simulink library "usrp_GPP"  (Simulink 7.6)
settings: Solver=ode45  SolverMode=SingleTasking  StartTime=0.0  StopTime=10.0  RelTol=1e-3
undefined symbols (not defined in the file or in its folder): Bit, Channels, Complex, Disabled, INT16, kB, kSps, Mbit, N, S, s, zwei

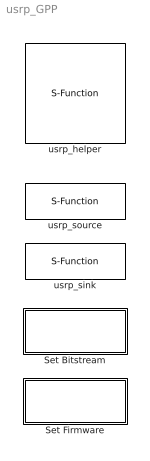
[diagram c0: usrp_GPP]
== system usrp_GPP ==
  Set Bitstream : Subsystem  mask{bitfile=zwei.rbf}
      mask prompts: bitfile "FPGA Bitfile"
  Set Firmware : Subsystem  mask{bitfile=zwei.rbf}
      mask prompts: bitfile "FPGA Bitfile"
  usrp_helper : S-Function  FunctionName=usrp_helper  EnableBusSupport=off  mask(USRP Helper){usrp_number=0, serial_number=S/N: 4556d9c1., daughterboards_rx=RX A: Flex 2400 Rx, RX B: WBX NG RX,, daughterboards_tx=TX A: Flex 2400 Tx, TX B: WBX NG TX., usb_block_size=0, usb_nblocks=0, firmware=C:\\Users\\nagel\\Documents\\sff_sdr\\Simulink-USRP\\simulink-usrp_2.1.0\\firmware\\rev4\\std.ihx, bitstream=C:\\Users\\nagel\\Documents\\sff_sdr\\Simulink-USRP\\simulink-usrp_2.1.0\\firmware\\rev4\\std_2rxhb_2tx.rbf, sample_time_factor=1}
      mask prompts: usrp_number "USRP Board Number:"; serial_number "Serial Number:"; daughterboards_rx "RX Daughterboards:"; daughterboards_tx "TX Daughterboards:"; usb_block_size "USB Block Size:"; usb_nblocks "USB Number of Blocks:"; firmware "Firmware Filename:"; bitstream "FPGA Bitstream Filename:"; sample_time_factor "Sample Time Factor:"
      mask help: Use this block to set common settings for a USRP device.
      mask init:
      | % Set default bitstream and firmware if not specified yet
      | bitstream_std_path = fullfile(usrpGetFirmwarePath(),'rev4','std_2rxhb_2tx.rbf');
      | firmware_std_path = fullfile(usrpGetFirmwarePath(),'rev4','std.ihx');
      | 
      | if strcmp(get_param(gcb,'firmware'),'')
      |     set_param(gcb,'firmware',firmware_std_path)
      | end
      |     
      | if strcmp(get_param(gcb,'bitstream'),'')
      |     set_param(gcb,'bitstream',bitstream_std_path)
      | end
  usrp_sink : S-Function  FunctionName=usrp_sink  Parameters=usrp_number,decimation,sample_width,vector_length,sideA_subdev1_datatype,sideA_subdev1_frequency,sideA_subdev1_frequency_port,sideA_subdev1_gain,sideB_subdev1_datatype,sideB_subdev1_frequency,sideB_subdev1_frequency_port,sideB_subdev1_gain, usrp_helper('GetParam', 'sample_time_factor'), usrp_helper('GetParam', 'usb_block_size'), usrp_helper('GetParam', 'usb_nblocks'), usrp_helper('GetParam', 'firm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  EnableBusSupport=off  mask(USRP Sink){usrp_number=0, serial_number=Unknown (USRP Board #0 not found)., decimation=512, sample_width=16 Bit, sampling_rate_and_bandwidth=1 Channels: 250 kSps, 976.563 kB/s, 7.62939 Mbit/s., vector_length=1024, sideA_subdev1_tab_=0, sideA_subdev1_subdevice=Unknown (USRP Board #0 not found)., sideA_subdev1_datatype=INT16 Complex, sideA_subdev1_frequency_range=Unknown., sideA_subdev1_frequency_port=off, sideA_subdev1_frequency=0, sideA_subdev1_gain_range=Unknown., sideA_subdev1_gain=0, sideB_subdev1_tab_=0, sideB_subdev1_subdevice=Unknown (USRP Board #0 not found)., sideB_subdev1_datatype=Disabled, sideB_subdev1_frequency_range=Unknown., sideB_subdev1_frequency_port=off, sideB_subdev1_frequency=0, sideB_subdev1_gain_range=Unknown., sideB_subdev1_gain=0}
      mask prompts: usrp_number "USRP Board Number:"; serial_number "Serial Number:"; decimation "Interpolation Factor:"; sample_width "Sample Width:"; sampling_rate_and_bandwidth "Effective Sampling Rate and Bandwidth:"; vector_length "Vector length:"; sideA_subdev1_tab_ "---------- Side A, Subdev 1: ----------"; sideA_subdev1_subdevice "Daughterboard / Subdevice:"; sideA_subdev1_datatype "Data Type:"; sideA_subdev1_frequency_range "Frequency Range (Hz):"; sideA_subdev1_frequency_port "Frequency Input Port"; sideA_subdev1_frequency "Frequency (Hz):"; sideA_subdev1_gain_range "Gain Range (dB):"; sideA_subdev1_gain "Gain (dB):"; sideB_subdev1_tab_ "---------- Side B, Subdev 1: ----------"; sideB_subdev1_subdevice "Daughterboard / Subdevice:"; sideB_subdev1_datatype "Data Type:"; sideB_subdev1_frequency_range "Frequency Range (Hz):"; sideB_subdev1_frequency_port "Frequency Input Port"; sideB_subdev1_frequency "Frequency (Hz):"; sideB_subdev1_gain_range "Gain Range (dB):"; sideB_subdev1_gain "Gain (dB):"
      mask help: This block writes streams of samples from Simulink into the Universal Software Radio Peripheral (USRP).
      mask init:
      | %%%% Initialize
      | mask_display = 'image(imread(''usrp_50.jpg''))';
      | count=1;
      | sideA_color = '''magenta''';
      | sideB_color = '''yellow''';
      | 
      | % Side A, collect information
      | sideA_enabled = ~strcmp(get_param(gcb,'sideA_subdev1_datatype'),'Disabled');
      | sideA_complex = ~isempty(findstr('Complex',get_param(gcb,'sideA_subdev1_datatype')));
      | sideA_frqport = strcmp(get_param(gcb,'sideA_subdev1_frequency_port'),'on');
      | 
      | % Side B, collect information
      | sideB_enabled = ~strcmp(get_param(gcb,'sideB_subdev1_datatype'),'Disabled');
      | sideB_complex = ~isempty(findstr('Complex',get_param(gcb,'sideB_subdev1_datatype')));
      | sideB_frqport = strcmp(get_param(gcb,'sideB_subdev1_frequency_port'),'on');
      | 
      | %%%% Check for Data Input-Ports
      | % Side A
      | if (sideA_enabled && sideA_complex)
      |     mask_display = [mask_display ';color(' sideA_color ');port_label(''input'', ' num2str(count) ', ''A IQ'')'];
      |     count = count + 1;
      | elseif (sideA_enabled && ~sideA_complex)
      |     mask_display = [mask_display ';color(' sideA_color ');port_label(''input'', ' num2str(count) ', ''A I'')'];
      |     mask_display = [mask_display ';color(' sideA_color ');port_label(''input'', ' num2str(count+1) ', ''A Q'')'];
      |     count = count + 2;
      | end
      | 
      | % Side B
      | if (sideB_enabled && sideB_complex)
      |     mask_display = [mask_display ';color(' sideB_color ');port_label(''input'', ' num2str(count) ', ''B IQ'')'];
      |     count = count + 1;
      | elseif (sideB_enabled && ~sideB_complex)
      |     mask_display = [mask_display ';color(' sideB_color ');port_label(''input'', ' num2str(count) ', ''B I'')'];
      |     mask_display = [mask_display ';color(' sideB_color ');port_label(''input'', ' num2str(count+1) ', ''B Q'')'];
      |     count = count + 2;
      | end
      | 
      | %%%% Check for dynamic Frequency Input-Ports
      | % Side A
      | if (sideA_frqport)
      |     mask_display = [mask_display ';color(' sideA_color ');port_label(''input'', ' num2str(count) ', ''A f'')'];
      |     count = count + 1;
      | end
      | 
      | % Side B
      | if (sideB_frqport)
      |     mask_display = [mask_display ';color(' sideB_color ');port_label(''input'', ' num2str(count) ', ''B f'')'];
      |     count = count + 1;
      | end
      | 
      | %%%% Set mask
      | set_param(gcb,'MaskDisplay',mask_display)
  usrp_source : S-Function  FunctionName=usrp_source  Parameters=usrp_number,decimation,sample_width,vector_length,sideA_subdev1_datatype,sideA_subdev1_frequency,sideA_subdev1_frequency_port,sideA_subdev1_gain,sideA_subdev1_antenna,sideA_subdev2_datatype,sideA_subdev2_frequency,sideA_subdev2_frequency_port,sideA_subdev2_gain,'',sideB_subdev1_datatype,sideB_subdev1_frequency,sideB_subdev1_frequency_port,sideB_subdev1_gain,sideB_subdev1_antenna,sideB_subdev2_data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  EnableBusSupport=off  mask(USRP Source){usrp_number=0, serial_number=Unknown (USRP Board #0 not found)., decimation=256, sample_width=16 Bit, sampling_rate_and_bandwidth=1 Channels: 250 kSps, 976.563 kB/s, 7.62939 Mbit/s., vector_length=1024, sideA_subdev1_tab_=0, sideA_subdev1_subdevice=Unknown (USRP Board #0 not found)., sideA_subdev1_datatype=INT16 Complex, sideA_subdev1_frequency_range=Unknown., sideA_subdev1_frequency_port=off, sideA_subdev1_frequency=0, sideA_subdev1_gain_range=Unknown., sideA_subdev1_gain=0, sideA_subdev1_antenna=Not applicable, sideA_subdev2_tab_=0, sideA_subdev2_subdevice=Unknown (USRP Board #0 not found)., sideA_subdev2_datatype=Disabled, sideA_subdev2_frequency_range=Unknown., sideA_subdev2_frequency_port=off, sideA_subdev2_frequency=0, sideA_subdev2_gain_range=Unknown., sideA_subdev2_gain=0, sideB_subdev1_tab_=0, sideB_subdev1_subdevice=Unknown (USRP Board #0 not found)., sideB_subdev1_datatype=Disabled, sideB_subdev1_frequency_range=Unknown., sideB_subdev1_frequency_port=off, sideB_subdev1_frequency=0, sideB_subdev1_gain_range=Unknown., sideB_subdev1_gain=0, sideB_subdev1_antenna=Not applicable, sideB_subdev2_tab_=, sideB_subdev2_subdevice=Unknown (USRP Board #0 not found)., sideB_subdev2_datatype=Disabled, sideB_subdev2_frequency_range=Unknown., sideB_subdev2_frequency_port=off, sideB_subdev2_frequency=0, sideB_subdev2_gain_range=Unknown., sideB_subdev2_gain=0}
      mask prompts: usrp_number "USRP Board Number:"; serial_number "Serial Number:"; decimation "Decimation Factor:"; sample_width "Sample Width:"; sampling_rate_and_bandwidth "Effective Sampling Rate and Bandwidth:"; vector_length "Vector length:"; sideA_subdev1_tab_ "---------- Side A, Subdev 1: ----------"; sideA_subdev1_subdevice "Daughterboard / Subdevice:"; sideA_subdev1_datatype "Data Type:"; sideA_subdev1_frequency_range "Frequency Range (Hz):"; sideA_subdev1_frequency_port "Frequency Input Port"; sideA_subdev1_frequency "Frequency (Hz):"; sideA_subdev1_gain_range "Gain Range (dB):"; sideA_subdev1_gain "Gain (dB):"; sideA_subdev1_antenna "Antenna:"; sideA_subdev2_tab_ "---------- Side A, Subdev 2: ---------"; sideA_subdev2_subdevice "Daughterboard / Subdevice:"; sideA_subdev2_datatype "Data Type:"; sideA_subdev2_frequency_range "Frequency Range (Hz):"; sideA_subdev2_frequency_port "Frequency Input Port"; sideA_subdev2_frequency "Frequency (Hz):"; sideA_subdev2_gain_range "Gain Range (dB):"; sideA_subdev2_gain "Gain (dB):"; sideB_subdev1_tab_ "---------- Side B, Subdev 1: ----------"; sideB_subdev1_subdevice "Daughterboard / Subdevice:"; sideB_subdev1_datatype "Data Type:"; sideB_subdev1_frequency_range "Frequency Range (Hz):"; sideB_subdev1_frequency_port "Frequency Input Port"; sideB_subdev1_frequency "Frequency (Hz):"; sideB_subdev1_gain_range "Gain Range (dB):"; sideB_subdev1_gain "Gain (dB):"; sideB_subdev1_antenna "Antenna:"; sideB_subdev2_tab_ "---------- Side B, Subdev 2: ----------"; sideB_subdev2_subdevice "Daughterboard / Subdevice:"; sideB_subdev2_datatype "Data Type:"; sideB_subdev2_frequency_range "Frequency Range (Hz):"; sideB_subdev2_frequency_port "Frequency Input Port"; sideB_subdev2_frequency "Frequency (Hz):"; sideB_subdev2_gain_range "Gain Range (dB):"; sideB_subdev2_gain "Gain (dB):"
      mask help: This block reads streams of samples from the Universal Software Radio Peripheral (USRP) into Simulink.
      mask init:
      | %%%% Initialize
      | mask_display = 'image(imread(''usrp_50.jpg''))';
      | count_input=1;
      | count_output=1;
      | sideA_color = '''magenta''';
      | sideB_color = '''yellow''';
      | 
      | % Side A Subdev 1, collect information
      | sideA1_enabled = ~strcmp(get_param(gcb,'sideA_subdev1_datatype'),'Disabled');
      | sideA1_complex = ~isempty(findstr('Complex',get_param(gcb,'sideA_subdev1_datatype')));
      | sideA1_frqport = strcmp(get_param(gcb,'sideA_subdev1_frequency_port'),'on');
      | 
      | % Side A Subdev 2, collect information
      | sideA2_enabled = ~strcmp(get_param(gcb,'sideA_subdev2_datatype'),'Disabled');
      | sideA2_complex = ~isempty(findstr('Complex',get_param(gcb,'sideA_subdev2_datatype')));
      | sideA2_frqport = strcmp(get_param(gcb,'sideA_subdev2_frequency_port'),'on');
      | 
      | % Side B Subdev 1, collect information
      | sideB1_enabled = ~strcmp(get_param(gcb,'sideB_subdev1_datatype'),'Disabled');
      | sideB1_complex = ~isempty(findstr('Complex',get_param(gcb,'sideB_subdev1_datatype')));
      | sideB1_frqport = strcmp(get_param(gcb,'sideB_subdev1_frequency_port'),'on');
      | 
      | % Side B Subdev 2, collect information
      | sideB2_enabled = ~strcmp(get_param(gcb,'sideB_subdev2_datatype'),'Disabled');
      | sideB2_complex = ~isempty(findstr('Complex',get_param(gcb,'sideB_subdev2_datatype')));
      | sideB2_frqport = strcmp(get_param(gcb,'sideB_subdev2_frequency_port'),'on');
      | 
      | %%%% Check for Data Output-Ports
      | % Side A Subdev 1
      | if (sideA1_enabled && sideA1_complex)
      |     mask_display = [mask_display ';color(' sideA_color ');port_label(''output'', ' num2str(count_output) ', ''A-1 IQ'')'];
      |     count_output = count_output + 1;
      | elseif (sideA1_enabled && ~sideA1_complex)
      |     mask_display = [mask_display ';color(' sideA_color ');port_label(''output'', ' num2str(count_output) ', ''A-1 I'')'];
      |     mask_display = [mask_display ';color(' sideA_color ');port_label(''output'', ' num2str(count_output+1) ', ''A-1 Q'')'];
      |     count_output = count_output + 2;
      | end
      | 
      | % Side A Subdev 2
      | if (sideA2_enabled && sideA2_complex)
      |     mask_display = [mask_display ';color(' sideA_color ');port_label(''output'', ' num2str(count_output) ', ''A-2 IQ'')'];
      |     count_output = count_output + 1;
      | elseif (sideA2_enabled && ~sideA2_complex)
      |     mask_display = [mask_display ';color(' sideA_color ');port_label(''output'', ' num2str(count_output) ', ''A-2 I'')'];
      |     mask_display = [mask_display ';color(' sideA_color ');port_label(''output'', ' num2str(count_output+1) ', ''A-2 Q'')'];
      |     count_output = count_output + 2;
      | end
      | 
      | % Side B Subdev 1
      | if (sideB1_enabled && sideB1_complex)
      |     mask_display = [mask_display ';color(' sideB_color ');port_label(''output'', ' num2str(count_output) ', ''B-1 IQ'')'];
      |     count_output = count_output + 1;
      | elseif (sideB1_enabled && ~sideB1_complex)
      |     mask_display = [mask_display ';color(' sideB_color ');port_label(''output'', ' num2str(count_output) ', ''B-1 I'')'];
      |     mask_display = [mask_display ';color(' sideB_color ');port_label(''output'', ' num2str(count_output+1) ', ''B-1 Q'')'];
      |     count_output = count_output + 2;
      | end
      | 
      | % Side B Subdev 2
      | if (sideB2_enabled && sideB2_complex)
      |     mask_display = [mask_display ';color(' sideB_color ');port_label(''output'', ' num2str(count_output) ', ''B-2 IQ'')'];
      |     count_output = count_output + 1;
      | elseif (sideB2_enabled && ~sideB2_complex)
      |     mask_display = [mask_display ';color(' sideB_color ');port_label(''output'', ' num2str(count_output) ', ''B-2 I'')'];
      |     mask_display = [mask_display ';color(' sideB_color ');port_label(''output'', ' num2str(count_output+1) ', ''B-2 Q'')'];
      |     count_output = count_output + 2;
      | end
      | 
      | %%%% Check for dynamic Frequency Input-Ports
      | % Side A Subdev 1
      | if (sideA1_frqport)
      |     mask_display = [mask_display ';color(' sideA_color ');port_label(''input'', ' num2str(count_input) ', ''A-1 f'')'];
      |     count_input = count_input + 1;
      | end
      | 
      | % Side A Subdev 2
      | if (sideA2_frqport)
      |     mask_display = [mask_display ';color(' sideA_color ');port_label(''input'', ' num2str(count_input) ', ''A-2 f'')'];
      |     count_input = count_input + 1;
      | end
      | 
      | % Side B Subdev 1
      | if (sideB1_frqport)
      |     mask_display = [mask_display ';color(' sideB_color ');port_label(''input'', ' num2str(count_input) ', ''B-1 f'')'];
      |     count_input = count_input + 1;
      | end
      | 
      | % Side B Subdev 2
      | if (sideB2_frqport)
      |     mask_display = [mask_display ';color(' sideB_color ');port_label(''input'', ' num2str(count_input) ', ''B-2 f'')'];
      |     count_input = count_input + 1;
      | end
      | 
      | %%%% Set mask
      | set_param(gcb,'MaskDisplay',mask_display)

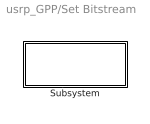
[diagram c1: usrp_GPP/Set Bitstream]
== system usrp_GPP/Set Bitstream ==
  Subsystem : Subsystem

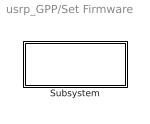
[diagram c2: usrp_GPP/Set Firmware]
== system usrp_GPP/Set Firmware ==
  Subsystem : Subsystem

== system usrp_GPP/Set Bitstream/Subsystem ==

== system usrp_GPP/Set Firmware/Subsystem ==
